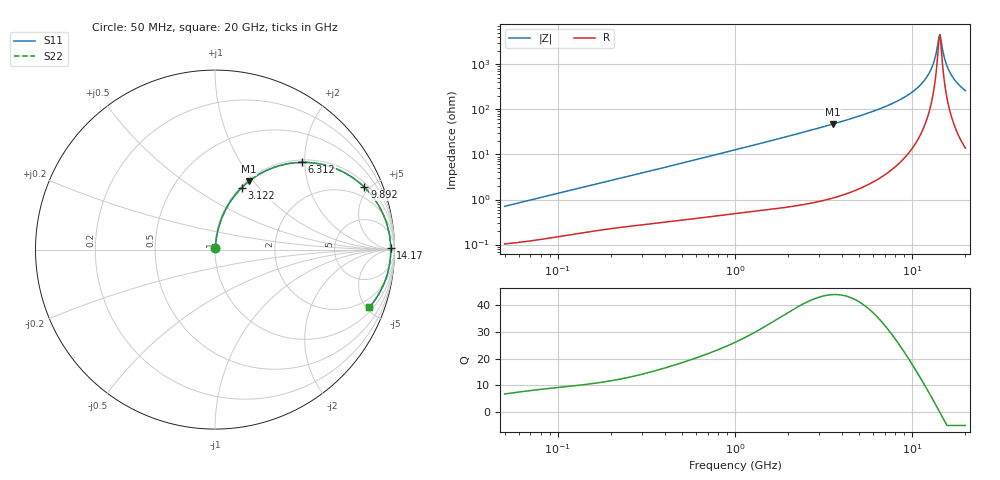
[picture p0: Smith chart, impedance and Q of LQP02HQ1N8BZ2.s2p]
!Murata Part Number: LQP02HQ1N8BZ2
!These Parameters are Measured in Series Mode Connection
!  o--[Z]--o
!Port1  Port2
!  o-------o
!Freq. Start=50[MHz] Stop=20[GHz], 401[Steps]
# Hz S RI R 50
!Freq.(Hz) S11(Real) S11(Imag) S21(Real) S21(Imag) S12(Real) S12(Imag) S22(Real) S22(Imag)
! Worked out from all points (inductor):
!   401 points, 50 MHz to 20 GHz, reference 50 ohm
!   read as one part in series: L = 2.21 nH near 51.52 MHz
!   highest Q = 43.9 at 3.572 GHz (marker M1), where L = 2.11 nH
!   self-resonance near 14.17 GHz
!   S11 on the Smith chart (normalised r, x): 50 MHz: 1.00, +0.01; 3.122 GHz: 1.02, +0.81; 6.312 GHz: 1.05, +1.94; 9.892 GHz: 1.25, +4.68; 14.17 GHz: 72, +41; 20 GHz: 1.28, -5.21
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5e7  0.00108 0.00697  0.9989 -0.00697  0.9989 -0.00697  0.00108 0.00697
1.364002e8  0.00214 0.0183  0.9979 -0.0183  0.9979 -0.0183  0.00214 0.0183
3.721004e8  0.0053 0.0476  0.9947 -0.0476  0.9947 -0.0476  0.0053 0.0476
1e9  0.0204 0.1233  0.9796 -0.1233  0.9796 -0.1233  0.0204 0.1233
2.728004e9  0.1161 0.3087  0.8839 -0.3087  0.8839 -0.3087  0.1161 0.3087
3.121702e9  0.1481 0.3439  0.8519 -0.3439  0.8519 -0.3439  0.1481 0.3439
3.572216e9  0.1886 0.38  0.8114 -0.38  0.8114 -0.38  0.1886 0.38
4.748272e9  0.3092 0.4504  0.6908 -0.4504  0.6908 -0.4504  0.3092 0.4504
6.311513e9  0.4863 0.486  0.5137 -0.486  0.5137 -0.486  0.4863 0.486
7.442007e9  0.6117 0.4711  0.3883 -0.4711  0.3883 -0.4711  0.6117 0.4711
9.892087e9  0.8329 0.3468  0.1671 -0.3468  0.1671 -0.3468  0.8329 0.3468
1.131968e10  0.9156 0.2394  0.0844 -0.2394  0.0844 -0.2394  0.9156 0.2394
1.238412e10  0.954 0.1534  0.046 -0.1534  0.046 -0.1534  0.954 0.1534
1.314879e10  0.9703 0.0917  0.0297 -0.0917  0.0297 -0.0917  0.9703 0.0917
1.396067e10  0.9784 0.0278  0.0216 -0.0278  0.0216 -0.0278  0.9784 0.0278
1.417136e10  0.9791 0.0116  0.0209 -0.0116  0.0209 -0.0116  0.9791 0.0116
1.438523e10  0.9792 -0.00453  0.0208 0.00453  0.0208 0.00453  0.9792 -0.00453
1.460232e10  0.9789 -0.0207  0.0211 0.0207  0.0211 0.0207  0.9789 -0.0207
1.550395e10  0.9721 -0.0848  0.0279 0.0848  0.0279 0.0848  0.9721 -0.0848
1.646126e10  0.9571 -0.1471  0.0429 0.1471  0.0429 0.1471  0.9571 -0.1471
1.800918e10  0.9203 -0.2342  0.0797 0.2342  0.0797 0.2342  0.9203 -0.2342
2e10  0.8594 -0.3221  0.1406 0.3221  0.1406 0.3221  0.8594 -0.3221
